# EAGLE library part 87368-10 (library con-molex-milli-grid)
RECEPTACAL
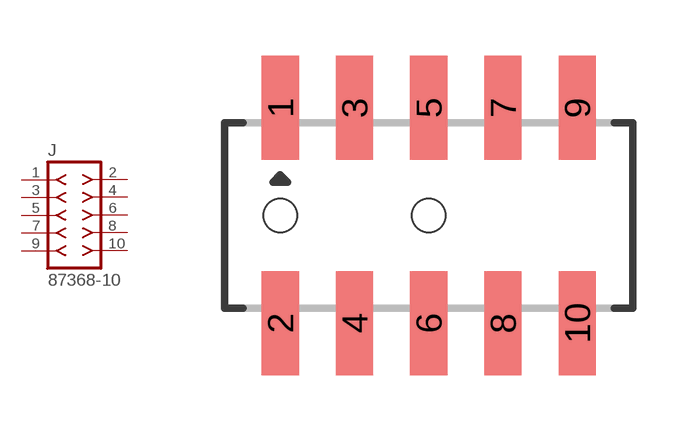
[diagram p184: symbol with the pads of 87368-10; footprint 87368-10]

Designator prefix J

## 87368-10  [87368-10]
1  1  pas
2  2  pas
3  3  pas
4  4  pas
5  5  pas
6  6  pas
7  7  pas
8  8  pas
9  9  pas
10  10  pas

## Footprint 87368-10 (pad centres in mm)
RECEPTACAL SMD Dual Row, Side Entry
smd 1 x 2.8: 1 -4,2.9; 2 -4,-2.9; 3 -2,2.9; 4 -2,-2.9; 5 0,2.9; 6 0,-2.9; 7 2,2.9; 8 2,-2.9; 9 4,2.9; 10 4,-2.9
hole 0.914 at -4,0
hole 0.914 at 0,0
